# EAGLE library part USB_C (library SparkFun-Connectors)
USB Type C 16Pin Connector Super Speed pins not available on the 16-pin purely SMD connector so this part is best for USB 2.0 implementations. D1 and D2 are tied together enabling D+/- no matter which way the cable is plugged into the connector. The two channel configuration pins (CC1/2) are exposed. These are normally connected to ground via 5.1k resistors but can be reconfigured for high current/high power applications.
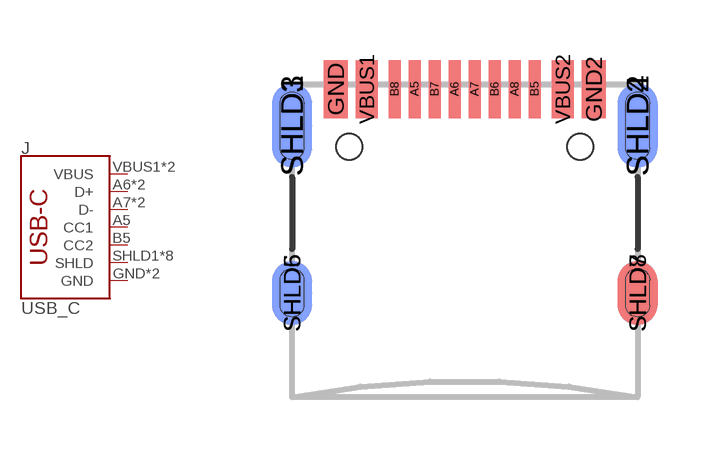
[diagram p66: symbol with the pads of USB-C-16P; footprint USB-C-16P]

Designator prefix J

## USB_C16PIN (PROD_ID: CONN-14122)  [USB-C-16P]
A5  CC1
A6  D+
A7  D-
B5  CC2
B6  D+
B7  D-
GND  GND
GND2  GND
SHLD1  SHLD
SHLD2  SHLD
SHLD3  SHLD
SHLD4  SHLD
SHLD5  SHLD
SHLD6  SHLD
SHLD7  SHLD
SHLD8  SHLD
VBUS1  VBUS
VBUS2  VBUS

## Footprint USB-C-16P (pad centres in mm)
smd 0.3 x 1.45: A5 -1.25,0; A6 -0.25,0; A7 0.25,0; A8 1.25,0; B5 1.75,0; B6 0.75,0; B7 -0.75,0; B8 -1.75,0
smd 0.6 x 1.45: GND -3.225,0; GND2 3.225,0
smd 1 x 2.1: SHLD1 -4.32,-0.915; SHLD2 4.32,-0.915
smd 1 x 2.1 bottom: SHLD3 -4.32,-0.915; SHLD4 4.32,-0.915
smd 1 x 1.6: SHLD5 -4.32,-5.095; SHLD8 4.32,-5.095
smd 1 x 1.6 bottom: SHLD6 -4.32,-5.095; SHLD7 4.32,-5.095
smd 0.55 x 1.45: VBUS1 -2.45,0; VBUS2 2.45,0
hole 0.65 at -2.89,-1.445
hole 0.65 at 2.89,-1.445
